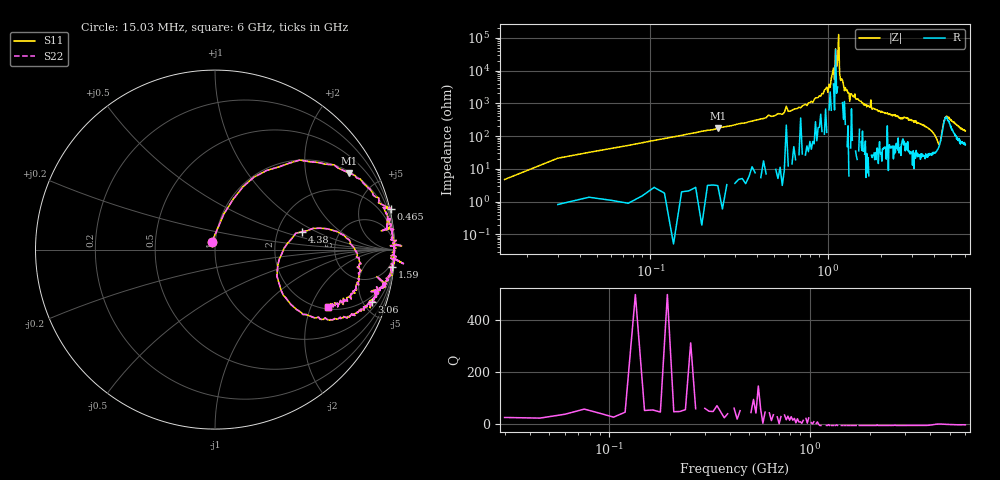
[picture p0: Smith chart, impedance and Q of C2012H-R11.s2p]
!	Network	Analyzer	HP8753E.07.74:	Oct	30	2002	Serial	No.	JP38451487
!	Hewlett-Packard
!	28	Aug	2009	10:39:51
!	Frequency	S11	S21	S12	S22
#	HZ	S	RI	R	50
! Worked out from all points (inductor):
!   400 points, 15.03 MHz to 6 GHz, reference 50 ohm
!   read as one part in series: L = 111 nH near 45.03 MHz
!   highest Q = 55.8 at 240 MHz (marker M1), where L = 114 nH
!   self-resonance near 1.095 GHz
!   S11 on the Smith chart (normalised r, x): 15.03 MHz: 0.96, +0.09; 465 MHz: -0.24, +8.70; 1.59 GHz: 2, -20; 3.06 GHz: 1.50, -5.73; 4.38 GHz: 2.75, +0.73; 6 GHz: 2.09, -2.68
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1.502992e7  -0.0166 0.0448  1.02 -0.0448  1.02 -0.0448  -0.0166 0.0448
3.002985e7  0.0496 0.199  0.95 -0.199  0.95 -0.199  0.0496 0.199
6.00297e7  0.156 0.35  0.844 -0.35  0.844 -0.35  0.156 0.35
2.400288e8  0.745 0.427  0.255 -0.427  0.255 -0.427  0.745 0.427
4.650277e8  0.98 0.228  0.0204 -0.228  0.0204 -0.228  0.98 0.228
1.020025e9  0.995 0.0256  0.00494 -0.0256  0.00494 -0.0256  0.995 0.0256
1.080025e9  0.997 0.00787  0.00278 -0.00787  0.00278 -0.00787  0.997 0.00787
1.095025e9  0.997 0.0186  0.00256 -0.0186  0.00256 -0.0186  0.997 0.0186
1.110024e9  0.998 -0.00061  0.00208 0.00061  0.00208 0.00061  0.998 -0.00061
1.125024e9  0.999 -0.00757  0.00125 0.00757  0.00125 0.00757  0.999 -0.00757
1.140024e9  0.999 -0.00482  0.000763 0.00482  0.000763 0.00482  0.999 -0.00482
1.155024e9  1 -0.000427  -0.00067 0.000427  -0.00067 0.000427  1 -0.000427
1.170024e9  1 -0.0123  -0.00024 0.0123  -0.00024 0.0123  1 -0.0123
1.245024e9  0.98 -0.0349  0.0202 0.0349  0.0202 0.0349  0.98 -0.0349
1.590022e9  0.987 -0.0982  0.0132 0.0982  0.0132 0.0982  0.987 -0.0982
2.01002e9  0.96 -0.169  0.0396 0.169  0.0396 0.169  0.96 -0.169
3.015015e9  0.89 -0.292  0.11 0.292  0.11 0.292  0.89 -0.292
3.060015e9  0.872 -0.293  0.128 0.293  0.128 0.293  0.872 -0.293
4.00501e9  0.548 -0.378  0.452 0.378  0.452 0.378  0.548 -0.378
4.380008e9  0.486 0.1  0.514 -0.1  0.514 -0.1  0.486 0.1
5.010005e9  0.798 -0.184  0.202 0.184  0.202 0.184  0.798 -0.184
6e9  0.631 -0.32  0.369 0.32  0.369 0.32  0.631 -0.32
